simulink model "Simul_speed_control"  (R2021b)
settings: Solver=ode1  StartTime=0.0  StopTime=5  FixedStep=0.002  RelTol=1e-3  AbsTol=1e-6  EnableMultiTasking=on
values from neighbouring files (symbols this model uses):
  K = 22.5    [test_your_model.m]
  T = 0.130    (= 0.13)    [test_your_model.m]

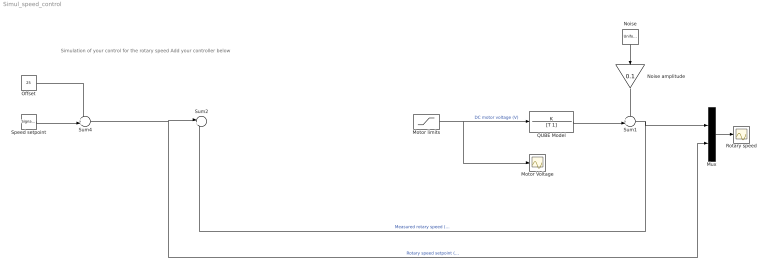
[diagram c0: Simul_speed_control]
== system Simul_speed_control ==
  note: Simulation of your control for the rotary speed Add your controller below
  Motor Voltage : Scope
  Motor limits : Saturate  UpperLimit=10  LowerLimit=-10
  Mux : Mux  Inputs=2
  Noise : UniformRandomNumber  SampleTime=0
  "Noise amplitude " : Gain  Gain=0.1
  Offset : Constant  Value=25
  QUBE Model : TransferFcn  Numerator=K  Denominator=[T 1]
  Rotary speed : Scope
  Speed setpoint : SignalGenerator  WaveForm=square  Amplitude=5  Frequency=0.2
  Sum1 : Sum  Inputs=++|
  Sum2 : Sum  Inputs=|+-
  Sum4 : Sum  Inputs=++|
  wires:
  Mux/1 -> Rotary speed/1
  Sum4/1 -> Sum2/1, Mux/2  "Rotary speed setpoint (rad/s)"
  "Noise amplitude "/1 -> Sum1/1
  QUBE Model/1 -> Sum1/2
  Sum1/1 -> Mux/1, Sum2/2  "Measured rotary speed (rad/s)"
  Noise/1 -> "Noise amplitude "/1
  Offset/1 -> Sum4/1
  Speed setpoint/1 -> Sum4/2
  Motor limits/1 -> QUBE Model/1, Motor Voltage/1  "DC motor voltage (V)"
  Sum2/1 -> ?
